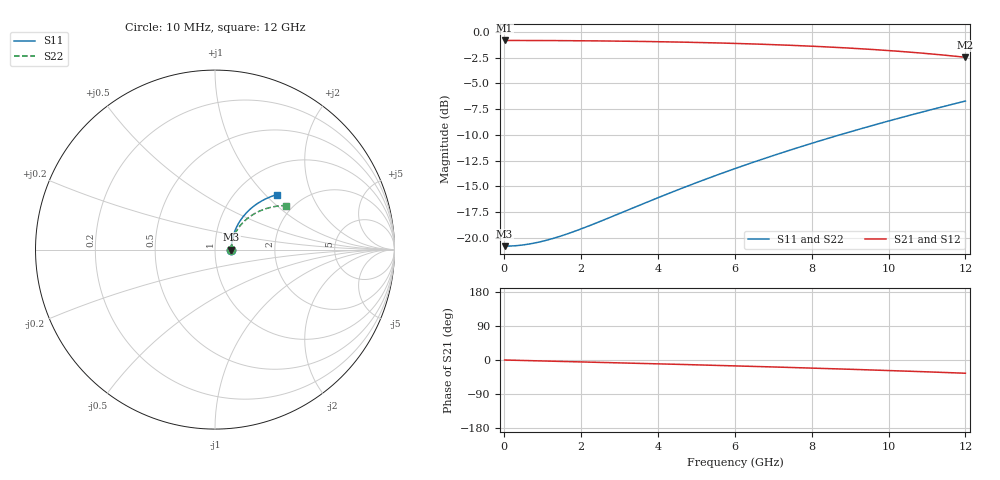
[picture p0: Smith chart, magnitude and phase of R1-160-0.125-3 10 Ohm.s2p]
!version-1
!date-03.2021
# MHz S RI R 50
!Freq ReS11 ImS11 ReS21 ImS21 ReS12 ImS12 ReS22 ImS22
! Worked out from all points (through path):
!   601 points, 10 MHz to 12 GHz, reference 50 ohm
!   highest |S21| = -0.83 dB at 10 MHz (marker M1); lowest = -2.5 dB at 12 GHz (marker M2)
!   group delay of S21, straight-line fit = 7.96 ps
!   lowest |S11| = -20.8 dB at 10 MHz (marker M3), VSWR 1.20, Z = 60 + j0.0326 ohm
!   |S11| at or under -10 dB: start of sweep to 8.737 GHz
!   |S22| runs from -20.8 to -6.7 dB; largest |S21 - S12| = 0
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10  0.0909 0.000269  0.9091 -0.000393  0.9091 -0.000393  0.0909 0.000258
230  0.091 0.0062  0.909 -0.00904  0.909 -0.00904  0.091 0.00593
450  0.0912 0.0121  0.9088 -0.0177  0.9088 -0.0177  0.0913 0.0116
670  0.0915 0.0181  0.9084 -0.0263  0.9084 -0.0263  0.0917 0.0173
910  0.092 0.0245  0.9078 -0.0358  0.9078 -0.0358  0.0923 0.0235
1150  0.0926 0.031  0.907 -0.0452  0.907 -0.0452  0.0932 0.0297
1410  0.0935 0.038  0.9059 -0.0554  0.9059 -0.0554  0.0943 0.0363
1690  0.0947 0.0456  0.9045 -0.0664  0.9045 -0.0664  0.0958 0.0435
2010  0.0962 0.0543  0.9026 -0.079  0.9026 -0.079  0.0979 0.0518
2430  0.0987 0.0656  0.8996 -0.0955  0.8996 -0.0955  0.1011 0.0625
3010  0.103 0.0814  0.8944 -0.1183  0.8944 -0.1183  0.1066 0.0773
4010  0.1127 0.1087  0.8827 -0.1575  0.8827 -0.1575  0.1192 0.1027
5010  0.1257 0.1362  0.8671 -0.1966  0.8671 -0.1966  0.1357 0.1275
6010  0.1422 0.1637  0.8474 -0.2354  0.8474 -0.2354  0.1566 0.1517
7030  0.1633 0.1916  0.8226 -0.2742  0.8226 -0.2742  0.1828 0.1751
8010  0.188 0.2179  0.7939 -0.3105  0.7939 -0.3105  0.213 0.196
9030  0.219 0.2442  0.7582 -0.3465  0.7582 -0.3465  0.2501 0.2153
10010  0.2544 0.2679  0.7181 -0.3785  0.7181 -0.3785  0.2915 0.2304
10530  0.2756 0.2794  0.6943 -0.3941  0.6943 -0.3941  0.3159 0.2367
11050  0.2985 0.2899  0.6687 -0.4085  0.6687 -0.4085  0.3419 0.2414
11570  0.3233 0.2994  0.6414 -0.4214  0.6414 -0.4214  0.3696 0.2445
12000  0.3451 0.3061  0.6174 -0.4308  0.6174 -0.4308  0.3937 0.2454
